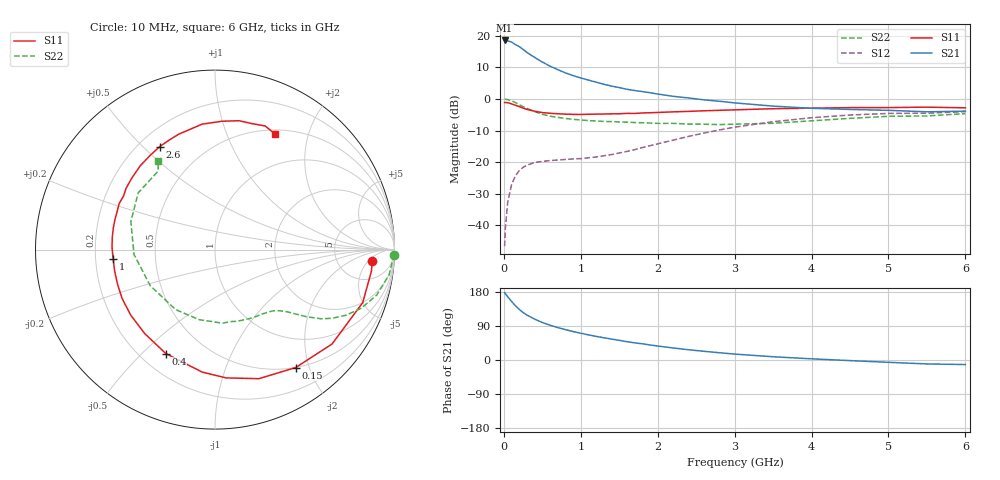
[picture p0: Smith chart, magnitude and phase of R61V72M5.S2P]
! SIEMENS Small Signal Semiconductors
! BFR193
! Si NPN RF Bipolar Junction Transistor in SOT23
! VCE = 1.75 V  IC = 2.5 mA
! Common Emitter S-Parameters:  May  1996
# GHz  S  MA  R  50
!  f  S11  S21  S12  S22
! GHz  MAG  ANG  MAG  ANG  MAG  ANG  MAG  ANG
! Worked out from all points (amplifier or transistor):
!   36 points, 10 MHz to 6 GHz, reference 50 ohm
!   highest |S21| = 18.5 dB at 10 MHz (marker M1)
!   |S21| within 3 dB of that: start of sweep to 258.6 MHz
!   unconditionally stable (mu >= 1): 1.087 GHz to 2.058 GHz
!   at 250 MHz: K = 0.27, MSG = 18.7 dB, |S12| = -21.6 dB
!   at 1.4 GHz: K = 1.11, MAG = 8.8 dB, |S12| = -17.6 dB
!   at 6 GHz: K = 0.99, MSG = 0.1 dB, |S12| = -4.0 dB
!   S11 on the Smith chart (normalised r, x): 10 MHz: 12, -6; 150 MHz: 0.50, -1.79; 400 MHz: 0.30, -0.59; 1 GHz: 0.27, -0.04; 2.6 GHz: 0.28, +0.56; 6 GHz: 0.55, +1.50
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0.01  0.8786 -4.0  8.437 177.8  0.0047 85.5  0.9971 -1.6
0.02  0.8798 -7.8  8.306 174.7  0.0091 84.7  0.9916 -3.3
0.05  0.8745 -19.7  8.306 167.0  0.0232 79.4  0.9806 -8.2
0.1  0.8378 -38.9  7.976 154.8  0.0438 69.8  0.9359 -15.7
0.15  0.7962 -55.6  7.257 143.2  0.0608 61.3  0.8785 -21.8
0.2  0.7597 -71.2  6.741 133.6  0.0736 54.7  0.8167 -26.6
0.25  0.7174 -85.1  6.087 125.3  0.0829 49.2  0.7565 -30.4
0.3  0.6861 -96.0  5.455 118.6  0.0896 45.3  0.7081 -33.0
0.4  0.6407 -115.3  4.559 108.0  0.0992 39.8  0.6313 -36.3
0.5  0.6102 -129.9  3.842 99.0  0.1031 36.7  0.5732 -38.7
0.6  0.5948 -142.1  3.316 91.9  0.1062 35.4  0.5353 -40.5
0.8  0.5765 -160.1  2.59 80.2  0.1105 35.7  0.4927 -43.7
1  0.5698 -175.0  2.152 70.6  0.1141 39.6  0.4655 -47.5
1.1  0.574 178.6  1.992 66.4  0.1175 42.0  0.4563 -50.0
1.3  0.5793 167.8  1.711 58.7  0.1266 47.1  0.4417 -54.7
1.6  0.5924 154.4  1.425 48.3  0.1482 54.1  0.4305 -63.3
2.2  0.6261 131.5  1.103 31.8  0.2234 59.6  0.4119 -84.5
2.6  0.6515 118.2  0.969 23.0  0.2888 57.1  0.4002 -102.5
3.5  0.7026 95.9  0.772 8.6  0.4374 42.5  0.4132 -150.9
4.5  0.7304 79.4  0.684 -1.6  0.5583 22.8  0.4941 161.6
5.5  0.7433 67.9  0.627 -10.4  0.5972 4.5  0.5396 126.1
6  0.7256 62.5  0.643 -12.0  0.6309 -0.7  0.5878 122.4
